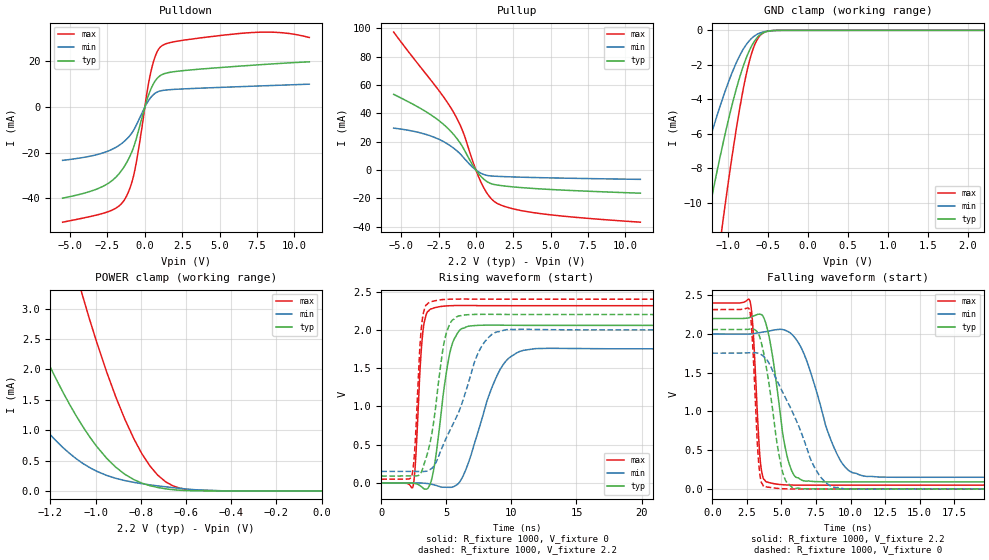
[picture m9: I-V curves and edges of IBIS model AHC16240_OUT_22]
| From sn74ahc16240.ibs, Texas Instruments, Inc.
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[Model]   AHC16240_OUT_22
Model_type  3-state
Enable   Active-Low
Vref =   0
Rref =   1000
Cref =   50p
Vmeas =   1.1
| variable   typ   min   max
C_comp   3.02pF   2.48pF   3.30pF
| C_pullup   3.95pF   2.61pF   4.81pF
| C_pulldown   3.97pF   3.08pF   5.11pF
| C_tri-state   3.02pF   2.48pF   3.30pF
[Temperature Range]   40   100   -40
| Ambient temperature   25   85   -40
[Voltage range]   2.2   2   2.4
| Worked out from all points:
|   slope of the pulldown table from 0 to 0.33 V, typ, clamps not added: 49.2 ohm
|   slope of the pullup table from 0 to 0.33 V, typ, clamps not added: 74.6 ohm
|   GND clamp passes 1 mA (typ) near -0.72 V on its own axis
|   POWER clamp passes 1 mA (typ) near -1.05 V on its own axis
|   rising waveform, R_fixture 1000, V_fixture 0: 20-80 % time 965ps typ, 2.03ns min, 435ps max; typ from 0 V to 2.06 V
|   falling waveform, R_fixture 1000, V_fixture 2.2: 20-80 % time 1ns typ, 1.96ns min, 412ps max; typ from 2.2 V to 0.092 V
|   rising waveform, R_fixture 1000, V_fixture 2.2: 20-80 % time 1.03ns typ, 2.45ns min, 429ps max; typ from 0.092 V to 2.2 V
|   falling waveform, R_fixture 1000, V_fixture 0: 20-80 % time 1.02ns typ, 2.52ns min, 382ps max; typ from 2.06 V to 0 V
[GND Clamp]
| AHC16240_OUT_22
|   Voltage   I(typ)   I(min)   I(max)
-5.5V     -169.3mA   -111.2mA   -212.8mA
-1.55V    -18.61mA   -11.75mA   -29.51mA
-1.495V   -17.08mA   -10.75mA   -27.27mA
-1.285V   -11.57mA   -7.16mA    -18.99mA
-1.26V    -10.95mA   -6.759mA   -18.04mA
-1.095V   -7.163mA   -4.284mA   -12.02mA
-1.055V   -6.319mA   -3.735mA   -10.64mA
-905mV    -3.486mA   -1.932mA   -5.865mA
-780mV    -1.657mA   -857.5uA   -2.655mA
-685mV    -720.6uA   -371.8uA   -1.018mA
-580mV    -187.8uA   -116.3uA   -205.7uA
2.2V      3.839nA    2.567nA    6.806nA
[POWER Clamp]
| AHC16240_OUT_22
|   Voltage   I(typ)   I(min)   I(max)
-5.5V     86.69mA    55.4mA     139.9mA
-1.62V    6.126mA    3.297mA    12.9mA
-1.585V   5.725mA    3.057mA    12.18mA
-1.34V    3.216mA    1.58mA     7.526mA
-1.18V    1.886mA    846.3uA    4.927mA
-1.055V   1.053mA    450.5uA    3.186mA
-950mV    534.8uA    254.5uA    1.952mA
-870mV    273.3uA    170.2uA    1.178mA
-795mV    128.8uA    119.3uA    613.6uA
-690mV    34.7uA     67.53uA    150.4uA
-555mV    1.82uA     18.6uA     8.944uA
-95.1fV   3.839nA    1.336nA    10.95nA
[Pulldown]
| AHC16240_OUT_22
|   Voltage   I(typ)   I(min)   I(max)
-5.5V     -39.97mA   -23.39mA   -50.51mA
-2.7V     -34.44mA   -19.89mA   -46.43mA
-1.815V   -29.92mA   -17.19mA   -43.83mA
-1.29V    -25.18mA   -14.53mA   -39.86mA
-935mV    -20.64mA   -11.97mA   -34.36mA
-660mV    -15.79mA   -9.071mA   -27.35mA
165mV     3.658mA    1.993mA    7.27mA
440mV     8.416mA    4.533mA    16.5mA
770mV     12.15mA    6.391mA    23.52mA
1.115V    14.12mA    7.201mA    26.76mA
7.195V    18.34mA    9.144mA    32.7mA
11V       19.84mA    10.04mA    30.51mA
[Pullup]
| AHC16240_OUT_22
|   Voltage   I(typ)   I(min)   I(max)
-5.5V     53.48mA    29.59mA    97.46mA
-3.185V   40.19mA    24.65mA    65.83mA
-2.285V   33.32mA    20.73mA    53.46mA
-1.56V    25.94mA    15.99mA    41.95mA
-870mV    15.97mA    9.306mA    27.2mA
-130mV    2.085mA    1.129mA    3.759mA
315mV     -4.252mA   -2.146mA   -8.042mA
770mV     -8.365mA   -3.863mA   -16.82mA
1.23V     -10.25mA   -4.356mA   -22.24mA
2.22V     -11.65mA   -4.801mA   -26.7mA
3.995V    -13.15mA   -5.332mA   -30.34mA
11V       -16.39mA   -6.617mA   -36.87mA
[Ramp]
| AHC16240_OUT_22
| variable   typ   min   max
dV/dt_r   1.28/1.01E-09   1.09/2.16E-09   1.43/4.56E-10
dV/dt_f   1.30/1.09E-09   1.15/2.16E-09   1.44/4.35E-10
R_load = 1000
[Rising Waveform]
| AHC16240_OUT_22
R_fixture =   1000
C_fixture =   0
L_fixture =   0
V_fixture =   0
V_fixture_min = 0
V_fixture_max = 0
|   Time   V(typ)   V(min)   V(max)
0s        172.7pV    466pV      60.18pV
2.42ns    -1.864mV   552.9uV    -55.63mV
2.615ns   -6.17mV    728.7uV    246mV
3.215ns   -66.34mV   -1.196mV   2.004V
4.1ns     249mV      -25.85mV   2.289V
5.315ns   1.734V     -56.13mV   2.315V
6.705ns   2.048V     267.8mV    2.317V
8.985ns   2.061V     1.435V     2.316V
10.93ns   2.059V     1.733V     2.315V
50ns      2.058V     1.753V     2.315V
[Falling Waveform]
| AHC16240_OUT_22
R_fixture =   1000
C_fixture =   0
L_fixture =   0
V_fixture =   2.2
V_fixture_min = 2
V_fixture_max = 2.4
|   Time   V(typ)   V(min)   V(max)
0s        2.2V       2V         2.4V
2.735ns   2.215V     2V         2.42V
2.96ns    2.231V     2.005V     2.016V
3.46ns    2.255V     2.019V     380.2mV
3.935ns   2.097V     2.033V     89.38mV
5.405ns   425.5mV    2.038V     51.58mV
6.625ns   103.6mV    1.746V     49.09mV
9.015ns   89.93mV    452.3mV    49.66mV
10.93ns   90.79mV    167.5mV    49.92mV
50ns      91.59mV    151.9mV    49.94mV
[Rising Waveform]
| AHC16240_OUT_22
R_fixture =   1000
C_fixture =   0
L_fixture =   0
V_fixture =   2.2
V_fixture_min = 2
V_fixture_max = 2.4
|   Time   V(typ)   V(min)   V(max)
0s        91.59mV    151.9mV    49.94mV
2.325ns   92.71mV    151.7mV    82.56mV
2.565ns   93.23mV    151.4mV    427.6mV
3.135ns   167.9mV    150.4mV    2.113V
3.935ns   697.5mV    199.7mV    2.372V
4.745ns   1.762V     491.4mV    2.396V
5.345ns   2.102V     711.9mV    2.401V
7.625ns   2.202V     1.759V     2.401V
9.44ns    2.202V     1.996V     2.4V
50ns      2.2V       2V         2.4V
[Falling Waveform]
| AHC16240_OUT_22
R_fixture =   1000
C_fixture =   0
L_fixture =   0
V_fixture =   0
V_fixture_min = 0
V_fixture_max = 0
|   Time   V(typ)   V(min)   V(max)
0s        2.058V     1.753V     2.315V
2.69ns    2.063V     1.758V     2.307V
2.91ns    2.064V     1.76V      1.877V
3.355ns   1.997V     1.749V     334mV
3.77ns    1.704V     1.701V     25.9mV
5.035ns   252.5mV    1.267V     3.59mV
5.94ns    7.746mV    937.2mV    -426.4uV
7.725ns   -66.54uV   181.6mV    -570.1uV
9.57ns    -769.5uV   954.8uV    -117.5uV
50ns      20.96nV    -16.33nV   27.9nV
